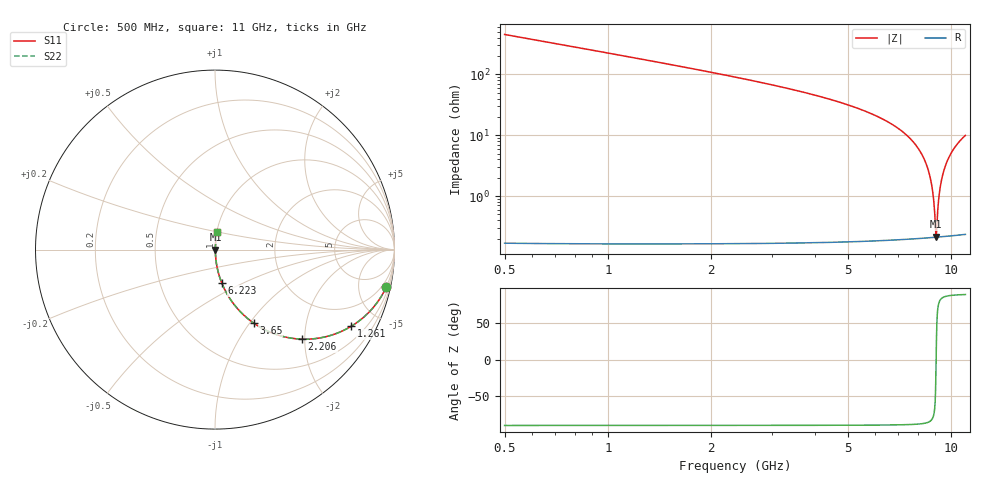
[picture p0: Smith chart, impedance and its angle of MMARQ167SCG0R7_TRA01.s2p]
! MMARQ167SCG0R7_TRA01  S-PARAMETER MODEL  ( General Type )
! Model Generated by TAIYO YUDEN Corporation (http://www.ty-top.com)
! Version 1.0
! TAIYO YUDEN Control No. 160201
! Copyright(c) 2016 TAIYO YUDEN CO.,LTD. All Rights Reserved.
! Product Description (link to TY-COMPAS)
! https://ds.yuden.co.jp/TYCOMPAS/or/detail?pn=MMARQ167SCG0R7BTRA01&u=M
! Products Name : Multilayer Ceramic Capacitors
! Characteristics :
!  Capacitance : 0.7 pF , Rated Voltage : 250V , TCC : CG / C0G
!  Case Size : 1.6 x 0.8 / 0.063 x 0.031 [mm/inch] , Thickness : 0.7 / 0.028 [mm/inch]
!  (Conditions: Temperature = 25 degC , DC Bias Current/Voltage = 0A / 0V)
! External Node Assignments :
!  1  o---| |---o  2
! GND o---------o GND
! Frequency Range : 500MHz  -  11000MHz  [ 401 STEP ]
# MHz S RI R 50
! Freq[MHz].  S11 Real  S11 Imag  S21 Real  S21 Imag  S12 Real  S12 Imag  S22 Real  S22 Imag
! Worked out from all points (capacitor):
!   401 points, 500 MHz to 11 GHz, reference 50 ohm
!   read as one part in series: C = 699 fF near 552.5 MHz
!   lowest |Z| = 216 mohm at 9.031 GHz (marker M1)
!   series resonance near 9.04 GHz, so ESL is about 440 pH
!   S11 on the Smith chart (normalised r, x): 500 MHz: 1.00, -9.08; 1.261 GHz: 1.00, -3.54; 2.206 GHz: 1.00, -1.94; 3.65 GHz: 1.00, -1.04; 6.223 GHz: 1.00, -0.39; 11 GHz: 1.00, +0.20
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500  0.9537 -0.2099  0.0463 0.2099  0.0463 0.2099  0.9537 -0.2099
841.25  0.878 -0.327  0.122 0.327  0.122 0.327  0.878 -0.327
1261.25  0.7581 -0.4278  0.2419 0.4278  0.2419 0.4278  0.7581 -0.4278
2206.25  0.4854 -0.4989  0.5146 0.4989  0.5146 0.4989  0.4854 -0.4989
2258.75  0.4721 -0.4984  0.5279 0.4984  0.5279 0.4984  0.4721 -0.4984
3650  0.2151 -0.4093  0.7849 0.4093  0.7849 0.4093  0.2151 -0.4093
4017.5  0.1725 -0.3759  0.8275 0.3759  0.8275 0.3759  0.1725 -0.3759
5750  0.0542 -0.2227  0.9458 0.2227  0.9458 0.2227  0.0542 -0.2227
6222.5  0.0374 -0.1851  0.9626 0.1851  0.9626 0.1851  0.0374 -0.1851
7508.75  0.0107 -0.0929  0.9893 0.0929  0.9893 0.0929  0.0107 -0.0929
8165  0.00463 -0.051  0.9954 0.051  0.9954 0.051  0.00463 -0.051
8585  0.00272 -0.0259  0.9973 0.0259  0.9973 0.0259  0.00272 -0.0259
8847.5  0.0022 -0.0108  0.9978 0.0108  0.9978 0.0108  0.0022 -0.0108
9005  0.0021 -0.00193  0.9979 0.00193  0.9979 0.00193  0.0021 -0.00193
9031.25  0.0021 -0.000467  0.9979 0.000467  0.9979 0.000467  0.0021 -0.000467
9083.75  0.00211 0.00244  0.9979 -0.00244  0.9979 -0.00244  0.00211 0.00244
9162.5  0.00216 0.00677  0.9978 -0.00677  0.9978 -0.00677  0.00216 0.00677
9267.5  0.00228 0.0125  0.9977 -0.0125  0.9977 -0.0125  0.00228 0.0125
9503.75  0.00278 0.0251  0.9972 -0.0251  0.9972 -0.0251  0.00278 0.0251
9845  0.00403 0.0428  0.996 -0.0428  0.996 -0.0428  0.00403 0.0428
10343.75  0.00684 0.0675  0.9932 -0.0675  0.9932 -0.0675  0.00684 0.0675
11000  0.0121 0.0981  0.9879 -0.0981  0.9879 -0.0981  0.0121 0.0981
